|//////////////////////////////////////////////////////////////////////////////
|//////////////////////////////////////////////////////////////////////////////
|   @@@@@@@   @@@@@@@   @@@@@@@   @@@@@@@   @@@@@@@   @@@@@@   @@
|   @@@@@@@@@   @@@@@@@@@   @@@@@@@@@   @@@@@@@@@   @@@@@@@@@ @@@@@@@@  @
|   @@@   @@@ @@@   @@@ @@@   @@@   @@@ @@@   @@@@   @@@  @
|   @@   @@ @@   @@ @@@@@@@@@@@ @@@@@@@@@@@ @@   @@   @@ @@
|   @@@   @@@ @@   @@   @@@ @@@   @@   @@   @@ @@
|   @@@@@@@@@  @@   @@  @@@@@@@@@   @@@@@@@@@  @@   @@   @@ @@
|   @@@@@@@   @@   @@   @@@@@@@   @@@@@@@   @@   @@   @@ @@
|   IBIS Model of MC74VHC1GT32
|   Single 2-Input OR Gate, TTL Level
|   Package Type: SC-74A, CASE 318BQ (DBV)
|   SC-88A/SC-70-5, CASE 419A-02 (DF)
|   SOT-953, CASE 527AE (P5)
|   SOT-553 (XV5), CASE 463B-01
|   UDFN6, CASE 517BX (1.00 x 1.00 mm)
|   UDFN6, CASE 517AA (1.20 x 1.00 mm)
|   UDFN6, CASE 517AQ (1.45 x 1.00 mm)
|   The model is covering the following Vccs:
|   2.0V, 2.5V, 3.3V, 5.0V
|//////////////////////////////////////////////////////////////////////////////
|//////////////////////////////////////////////////////////////////////////////
[IBIS Ver]   3.2
|   7.2 compatible
|//////////////////////////////////////////////////////////////////////////////
[Comment Char] |_char
|//////////////////////////////////////////////////////////////////////////////
[File Name]   74vhc1gt32_va_r0.ibs
|//////////////////////////////////////////////////////////////////////////////
[File Rev]   0.0
|   0.0 - February 07, 2025 - File created
|//////////////////////////////////////////////////////////////////////////////
[Date]   Feb 07, 2025
|//////////////////////////////////////////////////////////////////////////////
[Source]   From lab measurements and simulations at onsemi
|//////////////////////////////////////////////////////////////////////////////
[Notes]
   - The currents greater than +/- 100 mA are extrapolated
|//////////////////////////////////////////////////////////////////////////////
[Disclaimer]
   - onsemi Corporation hereby grants
   the user of this IBIS model a license to use this model
   under the following terms. This license is nonexclusive
   and nontransferable. Before using this IBIS model.
   After reading the terms and conditions of this license,
   the user either must accept these terms,
   or the IBIS model should be returned to onsemi within 30 days.
   - The user is hereby granted a license to use the IBIS model.
   This shall not be construed as a right to sell,
   or otherwise profit either by leasing or renting this software.
   - The user may modify the IBIS model to suit his specific
   applications but rights to derivative works and such
   modifications shall belong to onsemi.
   - This IBIS model is provided on an "as is" basis.
   onsemi makes absolutely no warranty with respect
   to the information contained herein.
   By use of this IBIS model, the user assumes full risk as to the
   quality and suitablility of the model to his particular use,
   and by using this model assumes the entire risk.
   Under all circumstances the user shall not hold
   onsemi liable in any way for the results obtained.
   onsemi reserves the right to make to improve
   the model for reliability, function, or design.
   onsemi does not convey any license under patent
   rights or any other intellectual property rights,
   including those of third parties.
   - onsemi is not obligated to provide maintenance
   or support for the licensed IBIS model.
   - Cont onsemi at ATTN:LOGIC APPLICATIONS/IBIS MODEL.
   5701 N Pima Rd, Scottsdale, AZ 85250
|//////////////////////////////////////////////////////////////////////////////
[Copyright]   (c) 2025 onsemi Corp.
|//////////////////////////////////////////////////////////////////////////////
|//////////////////////////////////////////////////////////////////////////////
[Component]   MC74VHC1GT32DBVT1G
|//////////////////////////////////////////////////////////////////////////////
[Manufacturer]  onsemi
|   Data Sheet:   MC74VHC1G32/D , Rev. 27,  Feb, 2024
|//////////////////////////////////////////////////////////////////////////////
[Package]
|   SC-74A
| DBV SUFFIX
| CASE 318BQ
| variable   typ   min   max
R_pkg   0.0710   0.0522   0.0935
L_pkg   1.2331nH   1.0634nH   1.4484nH
C_pkg   0.1280pF   0.1167pF   0.1367pF
|//////////////////////////////////////////////////////////////////////////////
[Pin]   signal_name   model_name   R_pin   L_pin   C_pin
1   B   In   0.0522   1.0634nH   0.1235pF
2   A   In   0.0588   1.1995nH   0.1367pF
3   GND   GND   0.0828   1.3327nH   0.1351pF
4   Y   Out   0.0935   1.4484nH   0.1279pF
5   VCC   POWER   0.0679   1.1215nH   0.1167pF
|//////////////////////////////////////////////////////////////////////////////
|//////////////////////////////////////////////////////////////////////////////
[Component]   MC74VHC1GT32DFT1G
|//////////////////////////////////////////////////////////////////////////////
[Manufacturer]  onsemi
|   Data Sheet:   MC74VHC1G32/D , Rev. 27,  Feb, 2024
|//////////////////////////////////////////////////////////////////////////////
[Package]
| SC-88A / SC-70-5
|   DF SUFFIX
|   CASE 419A-02
| variable   typ   min   max
R_pkg   0.0201   0.0170   0.0250
L_pkg   0.9982nH   0.8810nH   1.0690nH
C_pkg   0.1466pF   0.1187pF   0.2051pF
|//////////////////////////////////////////////////////////////////////////////
[Pin]   signal_name   model_name   R_pin   L_pin   C_pin
1   B   In   0.0191   1.0690nH   0.1625pF
2   A   In   0.0187   0.8810nH   0.1217pF
3   GND   GND   0.0170   1.0315nH   0.2051pF
4   Y   Out   0.0207   0.9600nH   0.1249pF
5   VCC   POWER   0.0250   1.0497nH   0.1187pF
|//////////////////////////////////////////////////////////////////////////////
|//////////////////////////////////////////////////////////////////////////////
[Component]   MC74VHC1GT32DFT2G
|//////////////////////////////////////////////////////////////////////////////
[Manufacturer]  onsemi
|   Data Sheet:   MC74VHC1G32/D , Rev. 27,  Feb, 2024
|//////////////////////////////////////////////////////////////////////////////
[Package]
R_pkg   0.0201   0.0170   0.0250
L_pkg   0.9982nH   0.8810nH   1.0690nH
C_pkg   0.1466pF   0.1187pF   0.2051pF
|//////////////////////////////////////////////////////////////////////////////
[Pin]   signal_name   model_name   R_pin   L_pin   C_pin
1   B   In   0.0191   1.0690nH   0.1625pF
2   A   In   0.0187   0.8810nH   0.1217pF
3   GND   GND   0.0170   1.0315nH   0.2051pF
4   Y   Out   0.0207   0.9600nH   0.1249pF
5   VCC   POWER   0.0250   1.0497nH   0.1187pF
|//////////////////////////////////////////////////////////////////////////////
|//////////////////////////////////////////////////////////////////////////////
[Component]   MC74VHC1GT32DFT1G-Q
|//////////////////////////////////////////////////////////////////////////////
[Manufacturer]  onsemi
|   Data Sheet:   MC74VHC1G32/D , Rev. 27,  Feb, 2024
|//////////////////////////////////////////////////////////////////////////////
[Package]
R_pkg   0.0201   0.0170   0.0250
L_pkg   0.9982nH   0.8810nH   1.0690nH
C_pkg   0.1466pF   0.1187pF   0.2051pF
|//////////////////////////////////////////////////////////////////////////////
[Pin]   signal_name   model_name   R_pin   L_pin   C_pin
1   B   In   0.0191   1.0690nH   0.1625pF
2   A   In   0.0187   0.8810nH   0.1217pF
3   GND   GND   0.0170   1.0315nH   0.2051pF
4   Y   Out   0.0207   0.9600nH   0.1249pF
5   VCC   POWER   0.0250   1.0497nH   0.1187pF
|//////////////////////////////////////////////////////////////////////////////
|//////////////////////////////////////////////////////////////////////////////
[Component]   MC74VHC1GT32DFT2G-Q
|//////////////////////////////////////////////////////////////////////////////
[Manufacturer]  onsemi
|   Data Sheet:   MC74VHC1G32/D , Rev. 27,  Feb, 2024
|//////////////////////////////////////////////////////////////////////////////
[Package]
R_pkg   0.0201   0.0170   0.0250
L_pkg   0.9982nH   0.8810nH   1.0690nH
C_pkg   0.1466pF   0.1187pF   0.2051pF
|//////////////////////////////////////////////////////////////////////////////
[Pin]   signal_name   model_name   R_pin   L_pin   C_pin
1   B   In   0.0191   1.0690nH   0.1625pF
2   A   In   0.0187   0.8810nH   0.1217pF
3   GND   GND   0.0170   1.0315nH   0.2051pF
4   Y   Out   0.0207   0.9600nH   0.1249pF
5   VCC   POWER   0.0250   1.0497nH   0.1187pF
|//////////////////////////////////////////////////////////////////////////////
|//////////////////////////////////////////////////////////////////////////////
[Component]   MC74VHC1GT32P5T5G
|//////////////////////////////////////////////////////////////////////////////
[Manufacturer]  onsemi
|   Data Sheet:   MC74VHC1G32/D , Rev. 27,  Feb, 2024
|//////////////////////////////////////////////////////////////////////////////
[Package]
|  SOT-953
| P5  SUFFIX
| CASE 527AE
| variable   typ   min   max
R_pkg   0.0786   0.0731   0.0817
L_pkg   1.1377nH   1.0330nH   1.1757nH
C_pkg   0.0487pF   0.0295pF   0.0642pF
|//////////////////////////////////////////////////////////////////////////////
[Pin]   signal_name   model_name   R_pin   L_pin   C_pin
1   A   In   0.0817   1.1757nH   0.0433pF
2   GND   GND   0.0731   1.0330nH   0.0295pF
3   B   In   0.0805   1.1531nH   0.0500pF
4   Y   Out   0.0789   1.1637nH   0.0642pF
5   VCC   POWER   0.0787   1.1630nH   0.0567pF
|//////////////////////////////////////////////////////////////////////////////
|//////////////////////////////////////////////////////////////////////////////
[Component]   MC74VHC1GT32MU1TCG
|//////////////////////////////////////////////////////////////////////////////
[Manufacturer]  onsemi
|   Data Sheet:   MC74VHC1G32/D , Rev. 27,  Feb, 2024
|//////////////////////////////////////////////////////////////////////////////
[Package]
|   UDFN-6
| 1.45 x 1.0
| CASE 517AQ
| variable   typ   min   max
R_pkg   0.0499   0.0010   0.0568
L_pkg   0.4063nH   0.0145nH   0.4786nH
C_pkg   0.1074pF   0.0765pF   0.1119pF
|//////////////////////////////////////////////////////////////////////////////
[Pin]   signal_name   model_name   R_pin   L_pin   C_pin
1   B   In   0.0568   0.4786nH   0.1119pF
2   A   In   0.0469   0.3812nH   0.1077pF
3   GND   GND   0.0541   0.4521nH   0.1099pF
4   Y   Out   0.0513   0.4206nH   0.1072pF
5   NC   NC   0.0010   0.0145nH   0.0765pF
6   VCC   POWER   0.0484   0.3921nH   0.1051pF
|//////////////////////////////////////////////////////////////////////////////
|//////////////////////////////////////////////////////////////////////////////
[Component]   MC74VHC1GT32MU2TCG
|//////////////////////////////////////////////////////////////////////////////
[Manufacturer]  onsemi
|   Data Sheet:   MC74VHC1G32/D , Rev. 27,  Feb, 2024
|//////////////////////////////////////////////////////////////////////////////
[Package]
|  UDFN-6
| 1.2 x 1.0
| CASE 517AA
| variable   typ   min   max
R_pkg   0.0380   0.0007   0.0502
L_pkg   0.3514nH   0.0262nH   0.4657nH
C_pkg   0.1033pF   0.0765pF   0.1113pF
|//////////////////////////////////////////////////////////////////////////////
[Pin]   signal_name   model_name   R_pin   L_pin   C_pin
1   B   In   0.0495   0.4460nH   0.1109pF
2   A   In   0.0407   0.3641nH   0.1069pF
3   GND   GND   0.0492   0.4551nH   0.1110pF
4   Y   Out   0.0502   0.4657nH   0.1113pF
5   NC   NC   0.0007   0.0262nH   0.0765pF
6   VCC   POWER   0.0461   0.4205nH   0.1085pF
|//////////////////////////////////////////////////////////////////////////////
|//////////////////////////////////////////////////////////////////////////////
[Component]   MC74VHC1GT32MU3TCG
|//////////////////////////////////////////////////////////////////////////////
[Manufacturer]  onsemi
|   Data Sheet:   MC74VHC1G32/D , Rev. 27,  Feb, 2024
|//////////////////////////////////////////////////////////////////////////////
[Package]
|  UDFN-6
| 1.0 x 1.0
| CASE 517BX
| variable   typ   min   max
R_pkg   0.0419   0.0344   0.0490
L_pkg   0.4237nH   0.3470nH   0.5107nH
C_pkg   0.1104pF   0.1061pF   0.1153pF
|//////////////////////////////////////////////////////////////////////////////
[Pin]   signal_name   model_name   R_pin   L_pin   C_pin
1   B   In   0.0421   0.4133nH   0.1099pF
2   A   In   0.0344   0.3470nH   0.1061pF
3   GND   GND   0.0443   0.4580nH   0.1121pF
4   Y   Out   0.0490   0.5107nH   0.1153pF
5   NC   NC   0.0004   0.0379nH   0.0765pF
6   VCC   POWER   0.0438   0.4489nH   0.1118pF
|//////////////////////////////////////////////////////////////////////////////
|//////////////////////////////////////////////////////////////////////////////
[Model Selector]   In
In_20   Vcc = 2.00
In_25   Vcc = 2.50
In_33   Vcc = 3.30
In_50   Vcc = 5.00
|//////////////////////////////////////////////////////////////////////////////
[Model Selector]   Out
Out_20   Vcc = 2.00
Out_25   Vcc = 2.50
Out_33   Vcc = 3.30
Out_50   Vcc = 5.00
| Models and submodels in the file (8): In_20 (Input), Out_20 (Output), In_25 (Input), Out_25 (Output), In_33 (Input), Out_33 (Output), In_50 (Input), Out_50 (Output)
